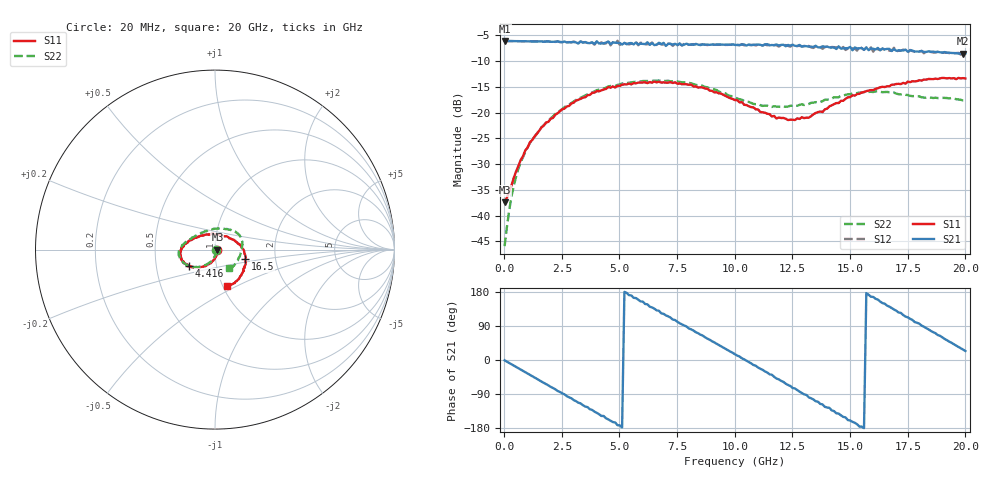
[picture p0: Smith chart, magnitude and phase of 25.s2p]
!Agilent Technologies,N5230A,US43500223,A.07.50.48
!Agilent N5230A: A.07.50.48
!Date: Saturday, October 10, 2015 14:46:51
!Correction: S11(Full 2 Port(1,2))
!S21(Full 2 Port(1,2))
!S12(Full 2 Port(1,2))
!S22(Full 2 Port(1,2))
!S2P File: Measurements: S11, S21, S12, S22:
# Hz S  RI  R 50
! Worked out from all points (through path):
!   201 points, 20 MHz to 20 GHz, reference 50 ohm
!   highest |S21| = -6.10 dB at 20 MHz (marker M1); lowest = -8.6 dB at 19.9 GHz (marker M2)
!   group delay of S21, straight-line fit = 96.4 ps
!   lowest |S11| = -37.4 dB at 20 MHz (marker M3), VSWR 1.03, Z = 51.4 - j0.0679 ohm
!   |S11| at or under -10 dB: start of sweep to end of sweep
!   |S22| runs from -45.9 to -13.8 dB; largest |S21 - S12| = 0.027
!   S11 on the Smith chart (normalised r, x): 20 MHz: 1.03, -0.00; 4.416 GHz: 0.74, -0.14; 16.5 GHz: 1.40, -0.15; 20 GHz: 1.05, -0.44
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2e7  0.0134 -0.000661  0.4952 -0.00735  0.4953 -0.00637  0.00497 -0.000897
4.196e8  0.0122 -0.0198  0.476 -0.1262  0.4768 -0.1267  0.00538 -0.0187
1.019e9  0.00121 -0.0457  0.3974 -0.2869  0.3972 -0.2869  -0.00556 -0.0456
2.3177e9  -0.0456 -0.0871  0.0709 -0.4841  0.0704 -0.4846  -0.0528 -0.0856
3.4166e9  -0.0955 -0.1014  -0.2337 -0.4156  -0.2437 -0.4114  -0.1049 -0.0964
4.4156e9  -0.1435 -0.0898  -0.4266 -0.2113  -0.417 -0.2137  -0.1497 -0.0887
5.7143e9  -0.1816 -0.0616  -0.4583 0.136  -0.464 0.1345  -0.1897 -0.0581
6.7133e9  -0.1967 -0.0313  -0.3041 0.3644  -0.3002 0.3614  -0.2027 -0.0283
7.6124e9  -0.1915 -0.00202  -0.0575 0.464  -0.0659 0.4598  -0.1982 -0.000354
8.3117e9  -0.1783 0.0189  0.1335 0.4438  0.1388 0.435  -0.1845 0.0188
1.001e10  -0.1157 0.0634  0.4376 0.1171  0.4369 0.1158  -0.1232 0.0687
1.09091e10  -0.0736 0.0781  0.4387 -0.1187  0.4303 -0.1223  -0.0784 0.0914
1.18082e10  -0.029 0.0825  0.3007 -0.3442  0.2987 -0.3363  -0.0351 0.1087
1.25075e10  0.00896 0.0847  0.127 -0.4372  0.13 -0.4327  -0.00397 0.1161
1.34066e10  0.0605 0.0745  -0.1041 -0.4196  -0.1008 -0.4105  0.0408 0.1178
1.43057e10  0.1105 0.0487  -0.3024 -0.3024  -0.2956 -0.3134  0.0845 0.1123
1.54046e10  0.1518 0.00637  -0.419 -0.0318  -0.4366 -0.0469  0.1289 0.0883
1.65035e10  0.1688 -0.0522  -0.3495 0.214  -0.3429 0.2179  0.151 0.0465
1.67033e10  0.1689 -0.0623  -0.3215 0.262  -0.3066 0.2536  0.1527 0.038
1.83017e10  0.1362 -0.1578  0.0402 0.385  0.0323 0.3917  0.1288 -0.0538
1.99001e10  0.0668 -0.2052  0.331 0.1707  0.3303 0.1696  0.0825 -0.1014
2e10  0.0664 -0.2031  0.342 0.1512  0.3397 0.1518  0.0794 -0.1032
